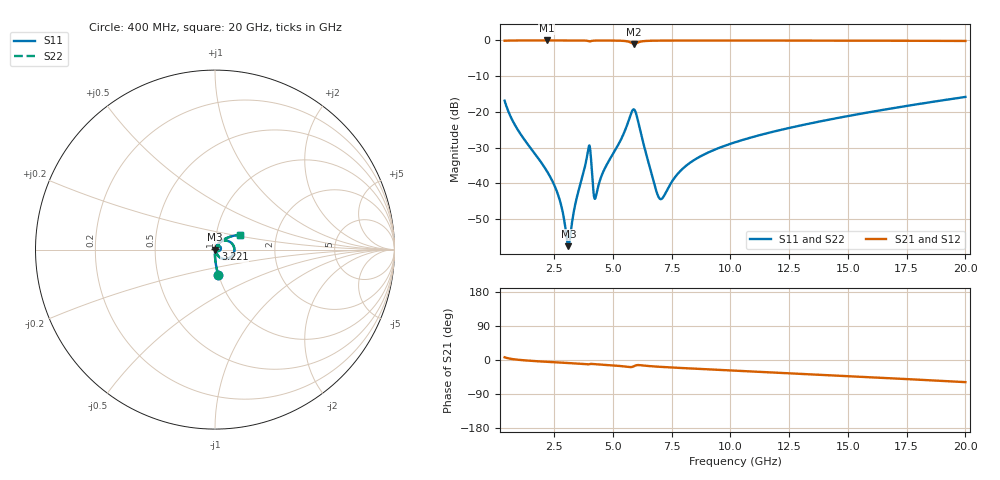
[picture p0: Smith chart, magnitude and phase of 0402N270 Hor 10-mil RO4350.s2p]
# GHz S MA R 50
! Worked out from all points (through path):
!   1960 points, 400 MHz to 20 GHz, reference 50 ohm
!   highest |S21| = -0.01 dB at 2.191 GHz (marker M1); lowest = -1.0 dB at 5.913 GHz (marker M2)
!   group delay of S21, straight-line fit = 8.35 ps
!   lowest |S11| = -57.6 dB at 3.111 GHz (marker M3), VSWR 1.00, Z = 50.1 - j0.0267 ohm
!   |S11| at or under -10 dB: start of sweep to end of sweep
!   |S22| runs from -57.6 to -15.8 dB; largest |S21 - S12| = 0
!   S11 on the Smith chart (normalised r, x): 400 MHz: 1.00, -0.29; 3.221 GHz: 1.00, +0.00; 20 GHz: 1.30, +0.22
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0.4  0.143 -82.6  0.9892 7.2  0.9892 7.2  0.143 -82.6
0.9502808  0.05674 -88.5  0.9976 0.8  0.9976 0.8  0.05674 -88.5
2.190914  0.01494 -91.0  0.9988 -4.8  0.9988 -4.8  0.01494 -91.0
2.721184  0.006173 -86.0  0.9987 -6.7  0.9987 -6.7  0.006173 -86.0
3.111383  0.001315 -11.7  0.9986 -8.0  0.9986 -8.0  0.001315 -11.7
3.22144  0.002169 41.8  0.9985 -8.4  0.9985 -8.4  0.002169 41.8
3.401531  0.005011 62.5  0.9983 -9.0  0.9983 -9.0  0.005011 62.5
3.671669  0.01111 66.9  0.9973 -10.1  0.9973 -10.1  0.01111 66.9
3.991833  0.0336 23.8  0.9722 -11.4  0.9722 -11.4  0.0336 23.8
4.061868  0.02502 -16.4  0.9749 -10.3  0.9749 -10.3  0.02502 -16.4
4.191935  0.006977 -7.2  0.9929 -10.8  0.9929 -10.8  0.006977 -7.2
4.281981  0.00653 36.1  0.9954 -11.3  0.9954 -11.3  0.00653 36.1
4.622154  0.01514 65.8  0.9967 -12.8  0.9967 -12.8  0.01514 65.8
5.912813  0.1076 -7.8  0.8932 -16.1  0.8932 -16.1  0.1076 -7.8
6.943338  0.006471 -24.4  0.9933 -17.8  0.9933 -17.8  0.006471 -24.4
7.12343  0.006233 11.8  0.9943 -18.4  0.9943 -18.4  0.006233 11.8
7.693721  0.01272 52.1  0.9958 -20.4  0.9958 -20.4  0.01272 52.1
8.304033  0.01953 58.3  0.9963 -22.3  0.9963 -22.3  0.01953 58.3
10.205  0.03749 57.8  0.9962 -28.1  0.9962 -28.1  0.03749 57.8
13.46667  0.06957 49.9  0.9943 -37.9  0.9943 -37.9  0.06957 49.9
16.73834  0.11 40.5  0.9903 -48.0  0.9903 -48.0  0.11 40.5
20  0.1617 30.4  0.9828 -58.4  0.9828 -58.4  0.1617 30.4
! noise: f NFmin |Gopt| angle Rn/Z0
0.4  0.001195  0.7753  1.303  0.001087
2.571  0.004412  0.6393  6.684  0.002302
4.752  0.01014  0.7005  12.17  0.006558
6.933  0.01734  0.7404  17.78  0.01307
9.104  0.0133  0.5963  23.02  0.005828
11.29  0.0143  0.553  28.14  0.00541
13.47  0.01582  0.5315  33.1  0.005517
15.64  0.01749  0.5195  37.87  0.005763
17.82  0.01923  0.5133  42.47  0.006073
20  0.02103  0.5113  46.88  0.006426
